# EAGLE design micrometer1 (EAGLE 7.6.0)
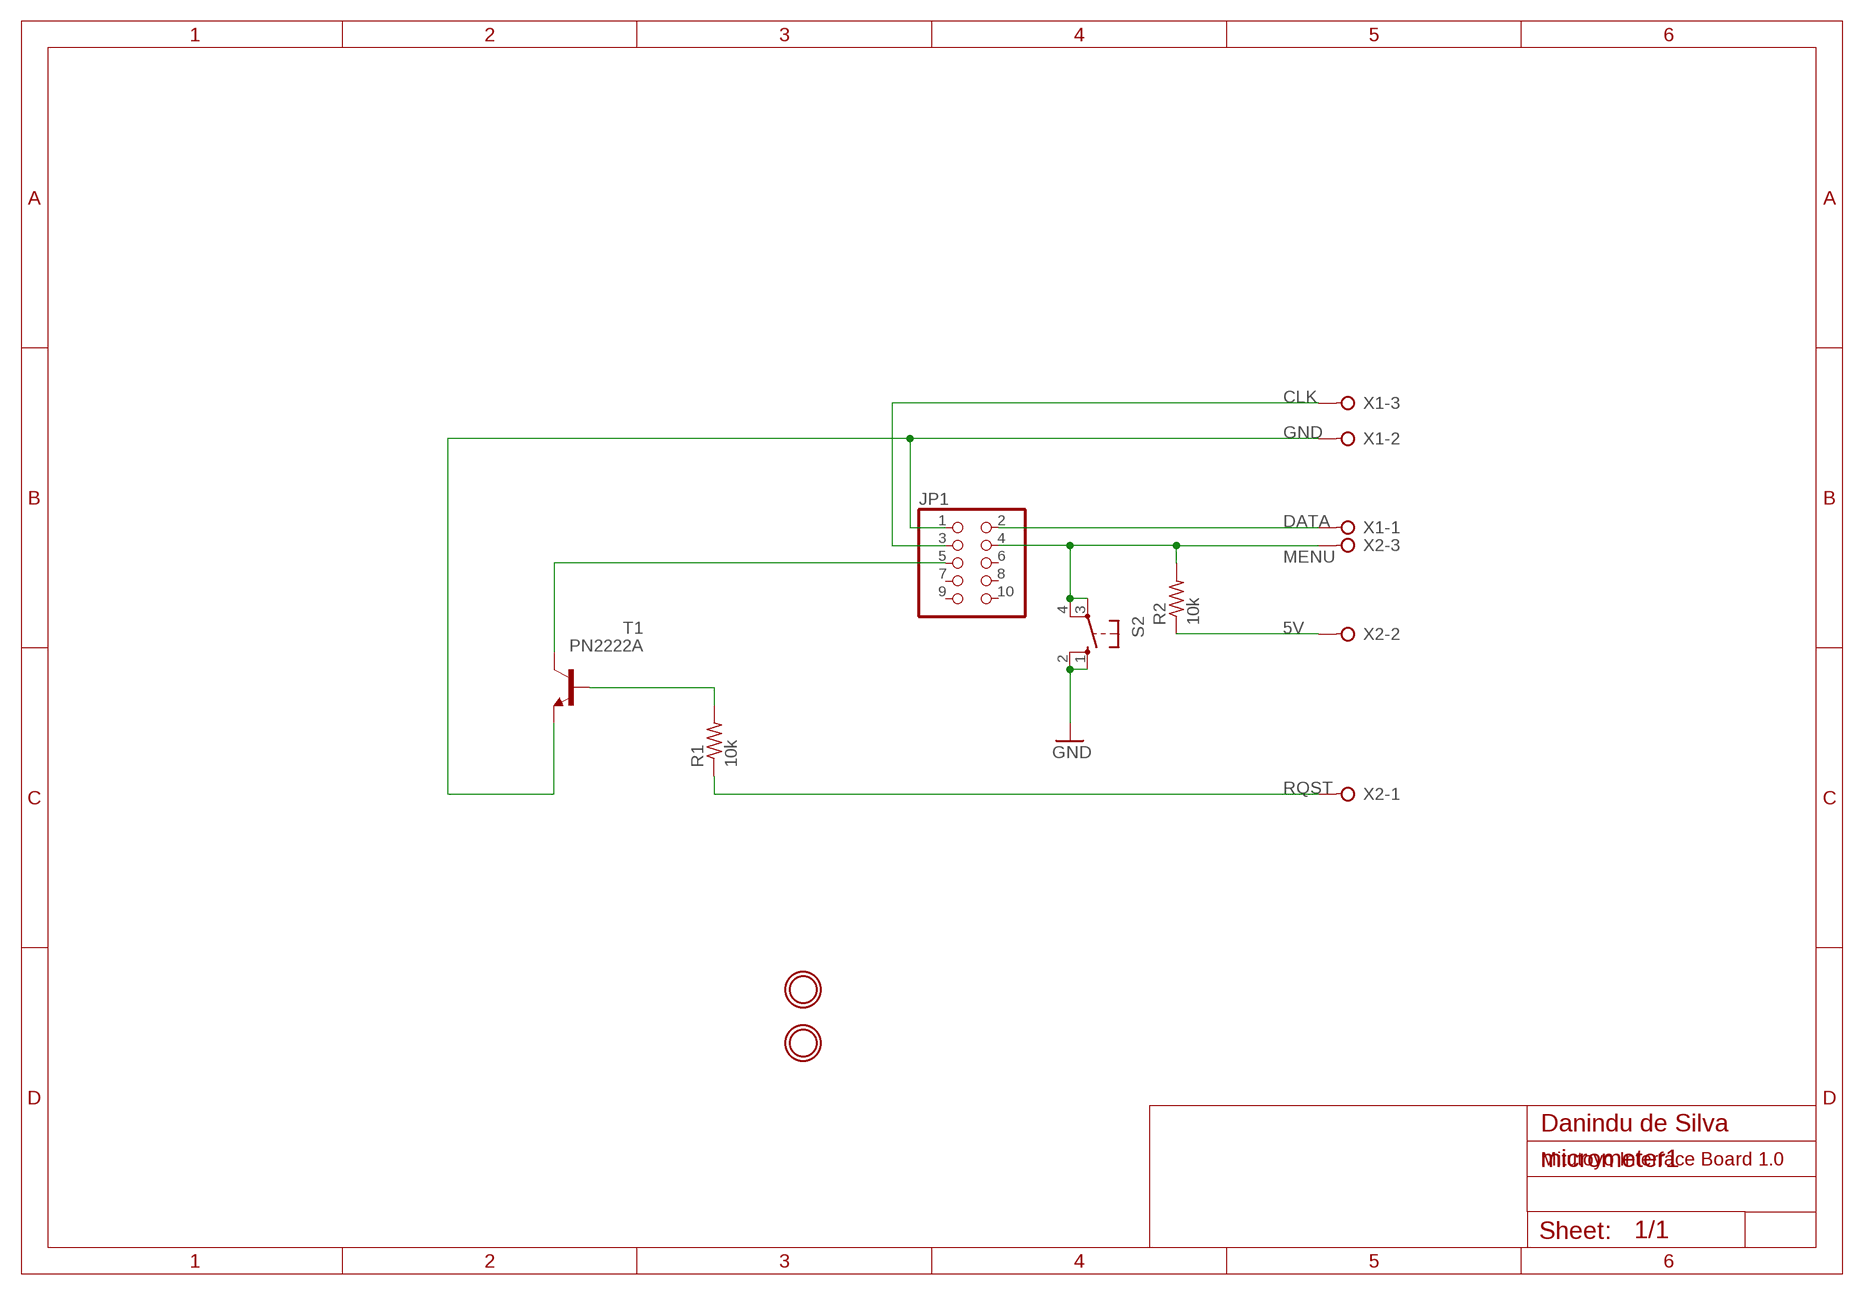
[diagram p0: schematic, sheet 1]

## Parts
JP1  PINHD-2X5SHROUDED  [2X05/90-SHROUDED]
R1  10k  R-US_0309/12  [0309/12]
R2  10k  R-US_0309/12  [0309/12]
S2  10-XX  [B3F-10XX]
T1  PN2222A  -NPN-TO92-EBC  [TO92-EBC]
U$1  MOUNTINGHOLE2.5  [MOUNTINGHOLE_2.5_PLATED]
U$2  MOUNTINGHOLE2.5  [MOUNTINGHOLE_2.5_PLATED]
X1  W237-3E  [W237-3E]
X2  W237-3E  [W237-3E]

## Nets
5V: R2.1 X2.2
CLK: JP1.3 X1.3
DATA: JP1.2 X1.1
GND: JP1.1 S2.1(S) S2.2(S1) T1.E X1.2
MENU: JP1.4 R2.2 S2.3(P) S2.4(P1) X2.3
N$1: R1.2 T1.B
N$8: JP1.5 T1.C
RQST: R1.1 X2.1
Unconnected: JP1.6 JP1.7 JP1.8 JP1.9 JP1.10

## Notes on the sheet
- Danindu de Silva
- Mitutoyo Interface Board 1.0

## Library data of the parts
JP1 = pinhead:PINHD-2X5: PIN HEADER
R1 R2 = resistor:R-US_: RESISTOR, American symbol
S2 = switch-omron:10-XX: OMRON SWITCH; MPN: B3F-1000; OC_FARNELL: 176432; OC_NEWARK: 36M3542
T1 = transistor-neu-to92:*-NPN-: NPN Transistror
U$1 U$2 = Adafruit SIM808 Breakout:MOUNTINGHOLE: Mounting Hole; BOM: EXCLUDE
X1 X2 = con-wago-508:W237-3E: WAGO SREW CLAMP; OC_FARNELL: unknown; OC_NEWARK: unknown

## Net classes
0 default: width 0.305 mm, drill 0.813 mm, clearance 0.305 mm

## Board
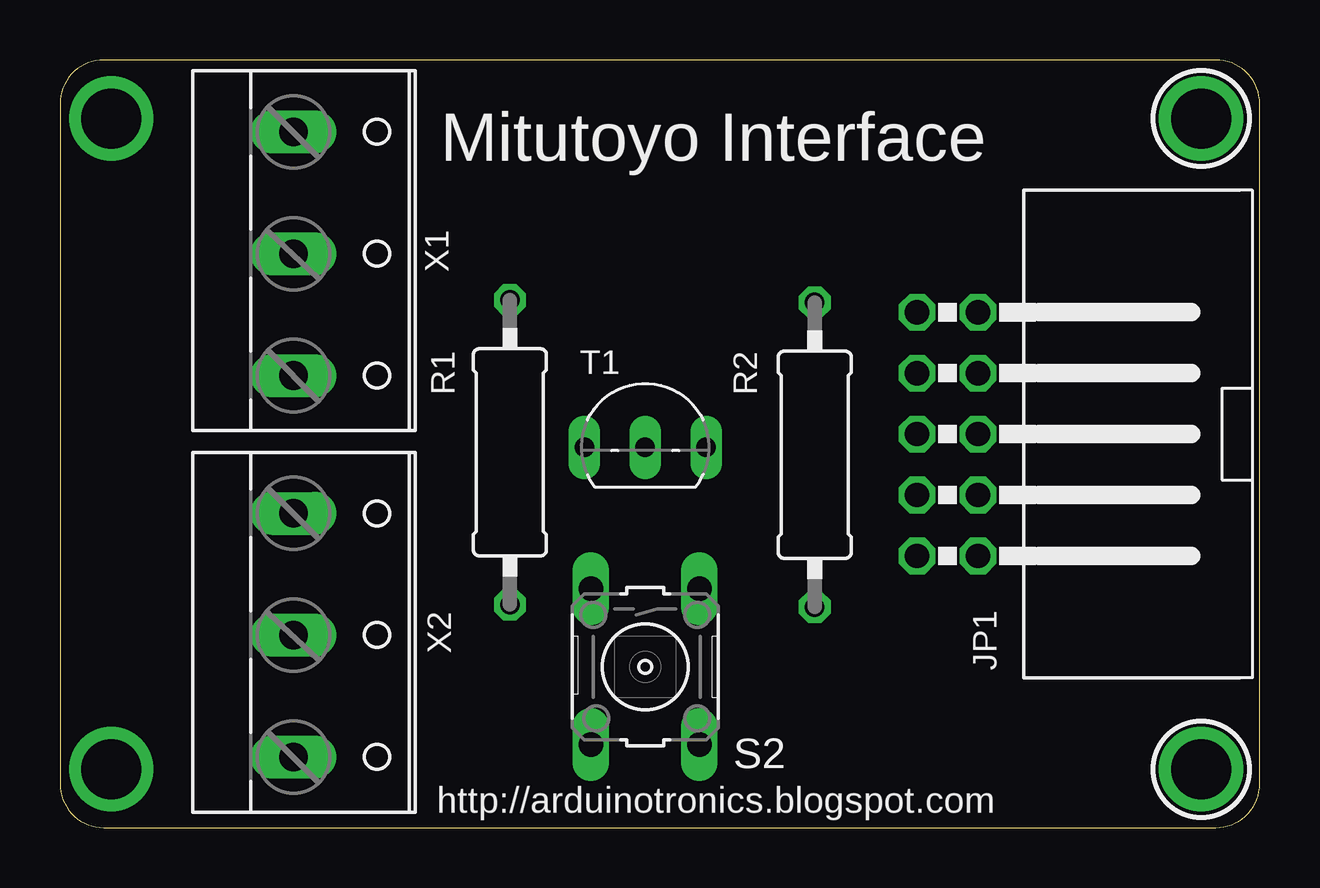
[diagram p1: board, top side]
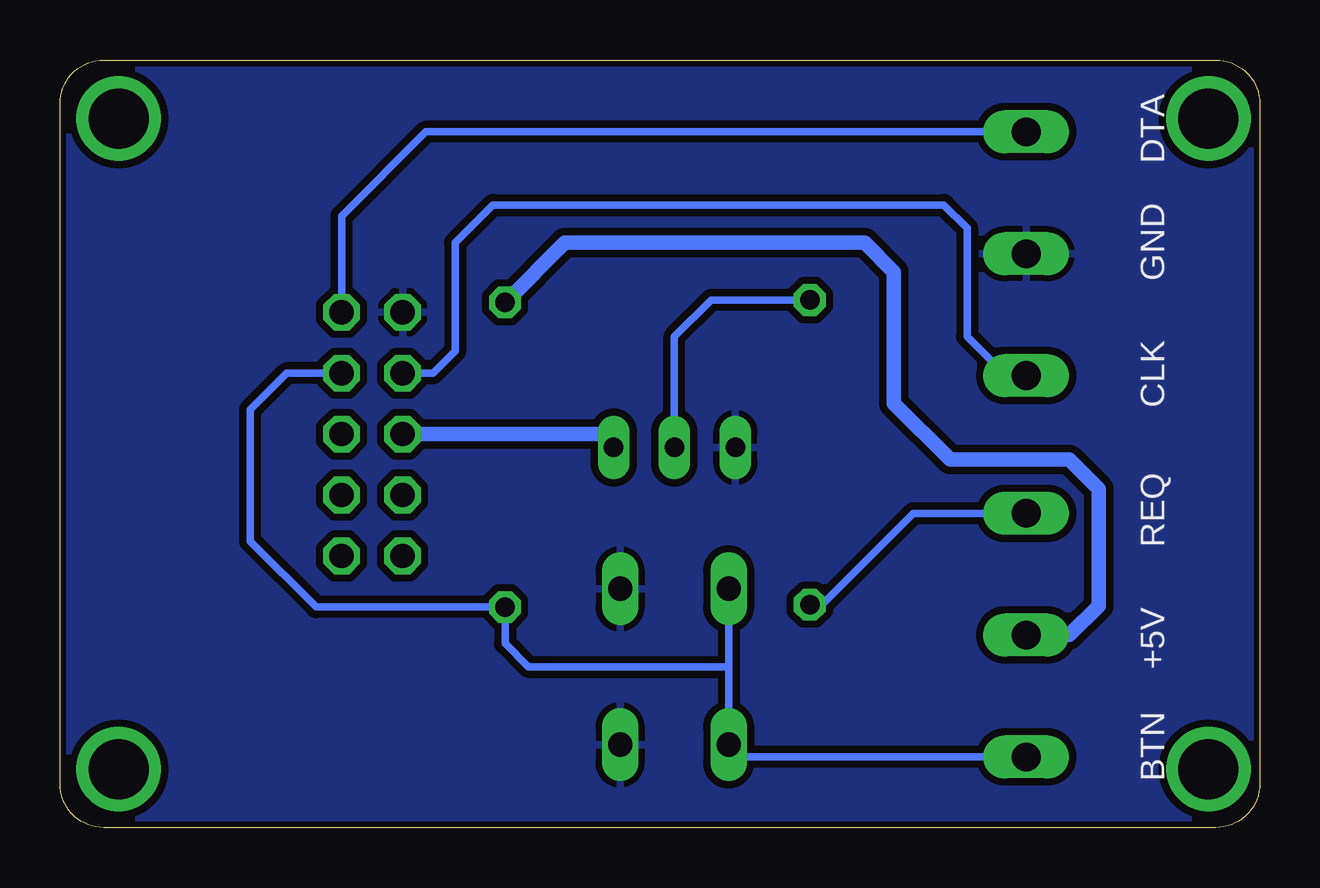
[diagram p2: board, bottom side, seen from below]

Size 49.99 x 32 mm. Coordinates in mm from the lower left corner, seen from the top.
Outline: 1.83,0 48.16,0 arc90 49.99,1.83 49.99,30.18 arc90 48.16,32 1.83,32 arc90 0,30.18 0,1.83 arc90 1.83,0
Copper layers (1*16): Top 0.035mm / dielectric 1.5mm / Bottom 0.035mm
Design rules "default *": minimum track width 10mil, minimum drill 24mil, track to track 8mil, track to pad 8mil, pad to pad 8mil, via to via 8mil, smd to smd 8mil, copper to edge 10mil, drill to drill 8mil, minimum pad ring 10mil, minimum via ring 8mil, stop-mask expansion 4mil, vias tented up to drill 0mil, thermal gap 10mil

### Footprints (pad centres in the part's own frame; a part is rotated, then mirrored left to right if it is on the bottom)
2X05/90-SHROUDED = drill 1.016 octagon: 1 -5.08,-10.16; 2 -5.08,-7.62; 3 -2.54,-10.16; 4 -2.54,-7.62; 5 0,-10.16; 6 0,-7.62; 7 2.54,-10.16; 8 2.54,-7.62; 9 5.08,-10.16; 10 5.08,-7.62
0309/12 = drill 0.813 octagon: 1 -6.35,0; 2 6.35,0
B3F-10XX = drill 1.016 long: 1 -3.251,2.261; 2 3.251,2.261; 3 -3.251,-2.261; 4 3.251,-2.261
TO92-EBC = drill 0.813 long: B 0,-1.27; C 2.54,-1.27; E -2.54,-1.27
MOUNTINGHOLE_2.5_PLATED = drill 2.5 pad 3.2: P$1 0,0
W237-3E = drill 1.194 long: 1 -5.08,-0.635; 2 0,-0.635; 3 5.08,-0.635

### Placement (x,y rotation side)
JP1  45.87,16.41 270 top
R1  18.75,15.65 90 top
R2  31.45,15.54 270 top
S2  24.38,6.71 270 top
T1  24.38,17.12 0 top
U$1  47.55,2.44 0 top
U$2  47.55,29.57 0 top
X1  10.36,23.93 270 top
X2  10.36,8.03 270 top

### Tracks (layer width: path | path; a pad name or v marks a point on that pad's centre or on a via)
5V
  Bottom 0.406: X2.2 7.92,8.03
  Bottom 0.61: 7.92,8.03 6.71,9.25 6.71,14.12 7.92,15.34 12.9,15.34 15.24,17.68 15.24,23.16 16.46,24.38 28.96,24.38 R2.1
CLK
  Bottom 0.305: JP1.3 34.44,18.95 33.53,19.86 33.53,24.38 31.95,25.96 13.16,25.96 12.19,24.99 12.19,20.47 10.57,18.85 X1.3
DATA
  Bottom 0.305: JP1.2 38.25,25.5 34.75,29.01 X1.1
GND
  pour Bottom: -0.61,32.31 50.6,32.31 50.6,-0.61 -0.61,-0.61
MENU
  Bottom 0.305: JP1.4 40.54,18.95 42.06,17.42 42.06,11.94 39.32,9.2 R2.2 31.45,7.67 30.48,6.71 22.12,6.71 | S2.3 22.12,6.71 | 22.12,6.71 S2.4 21.61,2.95 X2.3
N$1
  Bottom 0.305: R1.2 22.86,22 24.38,20.47 T1.B
N$2  (via drill 2.5 pad 3)
  other vias: 2.13,29.57
N$3  (via drill 2.5 pad 3)
  other vias: 2.13,2.44
N$8
  Bottom 0.61: JP1.5 27.48,16.41 T1.C
RQST
  Bottom 0.305: X2.1 14.43,13.11 18.24,9.3 R1.1

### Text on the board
tNames: Mitutoyo Interface | http://arduinotronics.blogspot.com
bNames: DTA | GND | CLK | REQ | +5V | BTN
